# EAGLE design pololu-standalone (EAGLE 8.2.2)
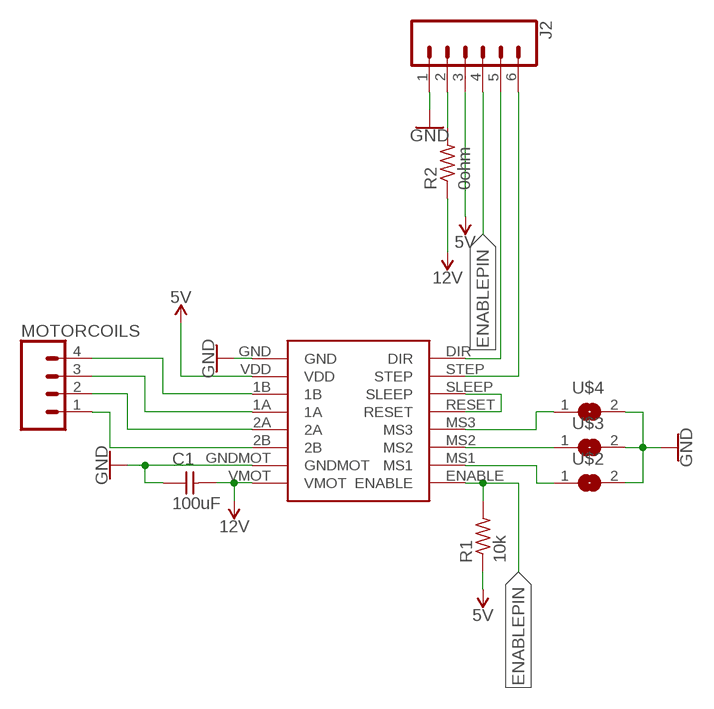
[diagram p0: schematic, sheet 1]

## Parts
C1  100uF  CAP-UNPOLARIZEDFAB  [C1206FAB]
J2  CONN_063.5MM-6  [SCREWTERMINAL-3.5MM-6]
MOTORCOILS  CONN_04SCREW  [SCREWTERMINAL-3.5MM-4]
POLOLU  POLOLUESTEPPERDRIVERDIL16MAT  [DIL16]
R1  10k  RES-US1206FAB  [R1206FAB]
R2  0ohm  RES-US1206FAB  [R1206FAB]
U$2  SOLDER_JUMPER  [SJFAB]
U$3  SOLDER_JUMPER  [SJFAB]
U$4  SOLDER_JUMPER  [SJFAB]

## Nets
5V: J2.3 POLOLU.VDD R1.1
12V: C1.2 POLOLU.VMOT R2.1
DIRPIN: J2.5 POLOLU.DIR
ENABLEPIN: J2.4 POLOLU.ENABLE R1.2
GND: C1.1 J2.1 POLOLU.GND POLOLU.GNDMOT U$2.2 U$3.2 U$4.2
N$1: POLOLU.RESET POLOLU.SLEEP
N$3: J2.2 R2.2
N$4: MOTORCOILS.1 POLOLU.2B
N$5: MOTORCOILS.2 POLOLU.2A
N$6: MOTORCOILS.3 POLOLU.1A
N$7: MOTORCOILS.4 POLOLU.1B
N$8: POLOLU.MS3 U$4.1
N$9: POLOLU.MS2 U$3.1
N$10: POLOLU.MS1 U$2.1
STEPPIN: J2.6 POLOLU.STEP

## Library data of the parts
C1 = 01fab:CAP-UNPOLARIZED
J2 = SparkFun-Connectors:CONN_06: Multi connection point. Often used as Generic Header-pin footprint for 0.1 inch spaced/style header connections On any of the 0.1 inch spaced packages, you can populate with these: Break Away Headers - Straight (PRT-00116) Break Away Male Headers - Right Angle (PRT-00553) Female Headers (PRT-00115)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
MOTORCOILS = SparkFun-Connectors:CONN_04: Multi connection point. Often used as Generic Header-pin footprint for 0.1 inch spaced/style header connections On any of the 0.1 inch spaced packages, you can populate with these: Break Away Headers - Straight (PRT-00116) Break Away Male Headers - Right Angle (PRT-00553) Female Headers (PRT-00115)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; PROD_ID: 2xCONN-08399; SF_ID: 2xPRT-08084
POLOLU = 01_reprap:POLOLUESTEPPERDRIVER: Pololu stepper driver based on the A4983.
R1 R2 = 01fab:RES-US: Resistor (US Symbol)
U$2-U$4 = 01fab:SOLDER_JUMPER

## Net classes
0 default: width 0.406 mm, drill 0.406 mm, clearance 0.406 mm
1 power: width 0.762 mm, drill 0.406 mm, clearance 0.406 mm

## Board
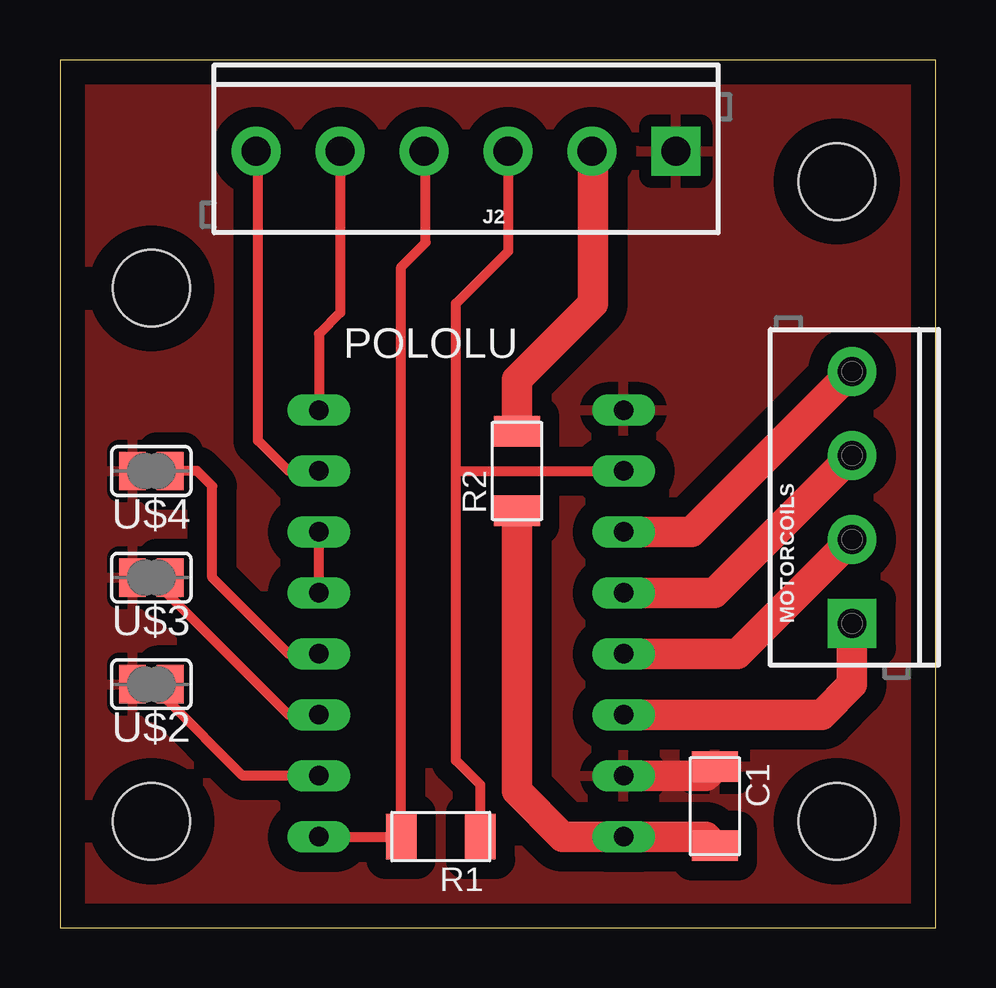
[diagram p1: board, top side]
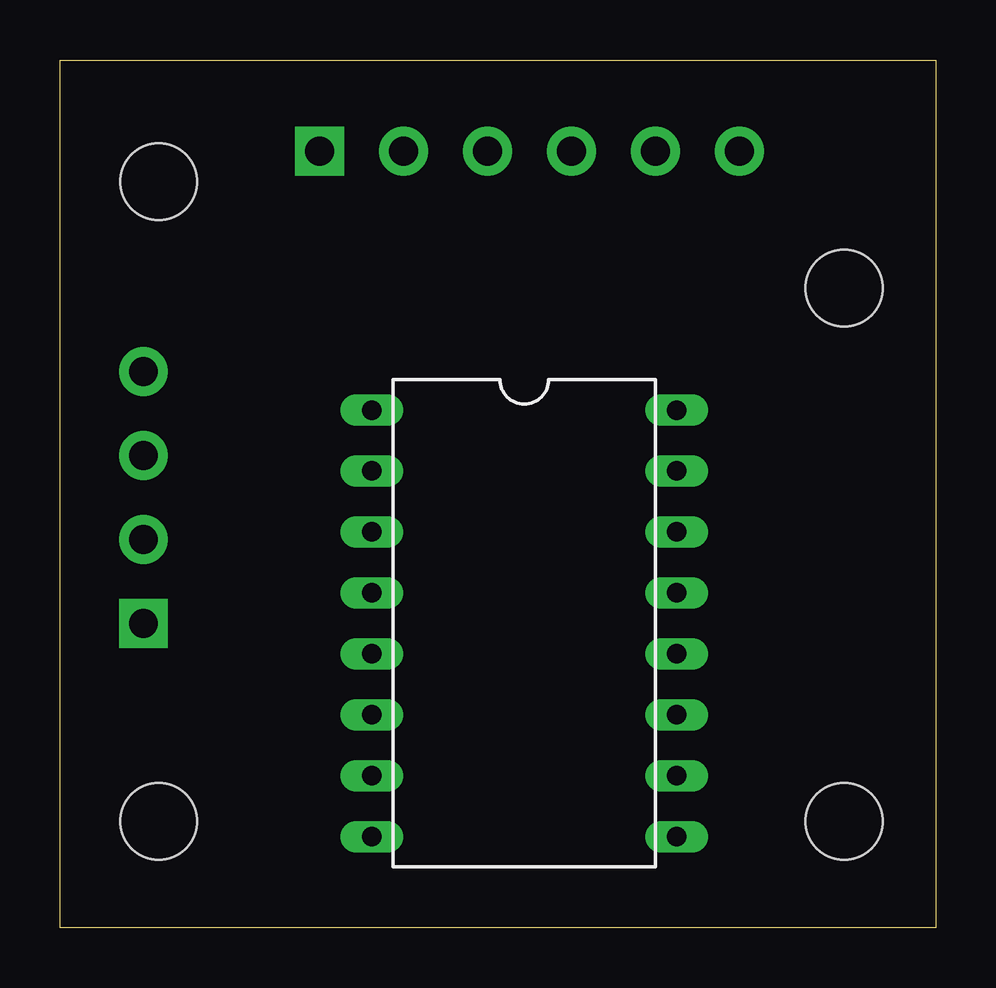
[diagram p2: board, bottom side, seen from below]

Size 36.5 x 36.19 mm. Coordinates in mm from the lower left corner, seen from the top.
Outline: 0,0 36.5,0 36.5,36.19 0,36.19 0,0
Copper layers (1*16): Top 0.035mm / dielectric 1.5mm / Bottom 0.035mm
Design rules "default *": minimum track width 12mil, minimum drill 0.35mm, track to track 16mil, track to pad 16mil, pad to pad 16mil, via to via 16mil, smd to smd 16mil, copper to edge 40mil, drill to drill 6mil, minimum pad ring 10mil, minimum via ring 8mil, stop-mask expansion 4mil, vias tented up to drill 0mil, thermal gap 20mil
Holes 3.2 mm at 32.38,4.45 32.38,31.11 3.81,26.67 3.81,4.45

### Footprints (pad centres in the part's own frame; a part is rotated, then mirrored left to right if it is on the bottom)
C1206FAB = smd 1.27 x 1.905: 1 -1.651,0; 2 1.651,0
SCREWTERMINAL-3.5MM-6 = drill 1.2 pad 2.032 square: 1 0,0 | drill 1.2 pad 2.032: 2 3.5,0; 3 7,0; 4 10.5,0; 5 14,0; 6 17.5,0
SCREWTERMINAL-3.5MM-4 = drill 1.2 pad 2.032 square: 1 0,0 | drill 1.2 pad 2.032: 2 3.5,0; 3 7,0; 4 10.5,0
DIL16 = drill 0.813 long: 1A -17.78,1.27; 1B -17.78,3.81; 2A -17.78,-1.27; 2B -17.78,-3.81; DIR -5.08,8.89; ENABLE -5.08,-8.89; GND -17.78,8.89; GNDMOT -17.78,-6.35; MS1 -5.08,-6.35; MS2 -5.08,-3.81; MS3 -5.08,-1.27; RESET -5.08,1.27; SLEEP -5.08,3.81; STEP -5.08,6.35; VDD -17.78,6.35; VMOT -17.78,-8.89
R1206FAB = smd 1.27 x 1.905: 1 -1.651,0; 2 1.651,0
SJFAB = smd 1.118 x 1.6: 1 -0.787,0; 2 0.787,0

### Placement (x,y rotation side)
C1  27.3,5.08 270 top
J2  25.68,32.38 180 top
MOTORCOILS  33.02,12.7 90 top
POLOLU  5.71,12.7 0 bottom
R1  15.88,3.81 180 top
R2  19.05,19.05 90 top
U$2  3.81,10.16 180 top
U$3  3.81,14.61 180 top
U$4  3.81,19.05 180 top

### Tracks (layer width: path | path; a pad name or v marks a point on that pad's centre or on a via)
5V
  Top 0.406: J2.3 18.68,28.2 16.51,26.04 16.51,19.05 | 16.51,19.05 POLOLU.VDD | R1.1 17.53,5.97 16.51,6.99 16.51,19.05
12V
  Top 1.27: C1.2 26.92,3.81 POLOLU.VMOT 20.95,3.81 19.05,5.71 R2.1
DIRPIN
  Top 0.406: J2.5 11.68,25.65 10.79,24.77 POLOLU.DIR
ENABLEPIN
  Top 0.406: POLOLU.ENABLE R1.2 14.22,27.56 15.24,28.57 15.24,32.33 J2.4
GND
  Top 1.27: POLOLU.GNDMOT 26.92,6.35 C1.1
  pour Top (isolate 0.813): -2.54,-1.91 40.01,-1.91 40.01,41.91 -2.54,41.91
N$1
  Top 0.406: POLOLU.RESET POLOLU.SLEEP
N$3
  Top 1.27: R2.2 19.05,22.86 22.23,26.04 22.23,32.34 J2.2
N$4
  Top 1.27: MOTORCOILS.1 33.02,10.16 31.75,8.89 POLOLU.2B
N$5
  Top 1.27: MOTORCOILS.2 31.58,14.76 31.57,14.76 28.25,11.43 POLOLU.2A
N$6
  Top 1.27: POLOLU.1A 27.29,13.97 MOTORCOILS.3
N$7
  Top 1.27: POLOLU.1B 26.33,16.51 MOTORCOILS.4
N$8
  Top 0.406: POLOLU.MS3 9.53,11.43 6.35,14.61 6.35,18.41 5.71,19.05 U$4.1
N$9
  Top 0.406: POLOLU.MS2 9.53,8.89 4.45,13.97 4.45,14.45 U$3.1
N$10
  Top 0.406: POLOLU.MS1 7.62,6.35 4.45,9.53 4.45,10.01 U$2.1
STEPPIN
  Top 0.406: POLOLU.STEP 9.53,19.05 8.26,20.32 8.26,32.31 J2.6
